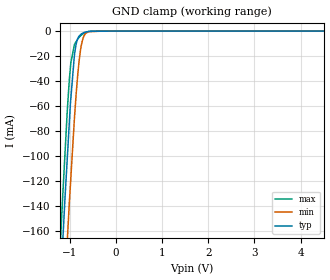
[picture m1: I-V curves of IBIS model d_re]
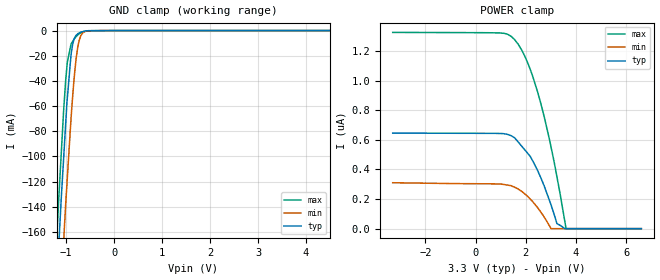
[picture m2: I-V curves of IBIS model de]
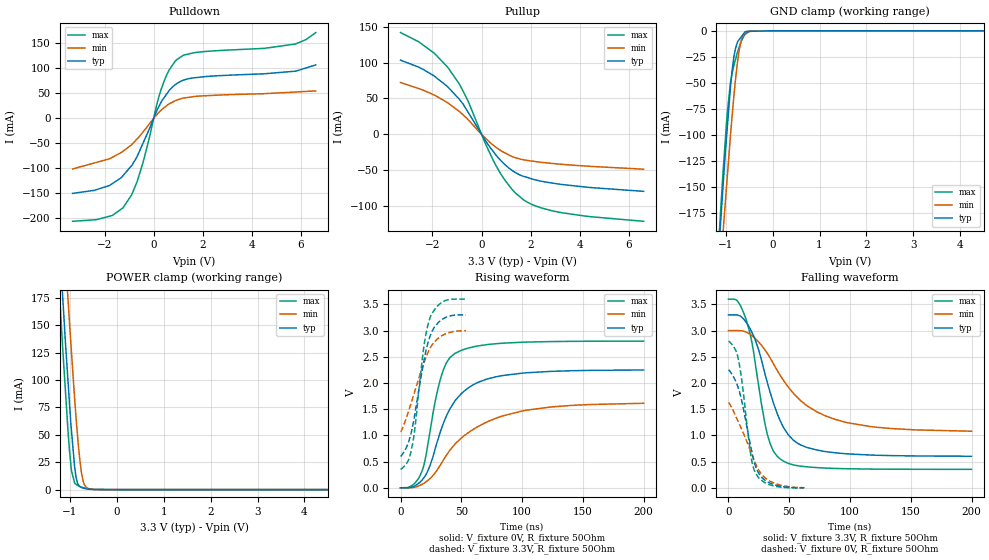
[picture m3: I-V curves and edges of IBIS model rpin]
|Texas Instruments Incorporated
| Robust Compact 3.3V-supply RS-485
| Marketing part#   Digital Voltage Range   Package-type   #pins
| SN65HVD72   3V - 3.6V   SOIC-8   8
[IBIS Ver]   3.2
[File name]   sn65hvd72.ibs
|SIMDE Ver   V3.0 - 201101 - RHL4 - Build 457
[File Rev]   1.0
[Date]   4/10/2012
[Source]
| Texas Instruments Incorporated.
| Analog-eLab Design Center, HPA
| 12500 TI Blvd
| Dallas, TX -75243
| e-mail: elab_scm_ibis@list.ti.com
[Notes]   Revision History:
| Rev 1.0: 4/10/2012
| - Initial version of the model
| - Model generated from simulations in TISPICE
| - Model matched to SPICE simulation
| - C_comp although listed in numerical order of value are
|   obtained from varying PVT conditions. For PVT conditions for
|   each specific value refer the buffer description under
|   respective [Model]. IBIS model user is responsible for using
|   appropriate C_comp to simulate for Signal Integrity.
|*  EXCEPTION:   *
|*  - For model d_re, there will be a leakage current in the GND   *
|*   clamp I-V Table because of the pullup on pad.   *
|*  - For model depin, there will be a leakage current in the POWER   *
|*   clamp I-V Table because of the pulldown on pad.   *
|*  - For model a_b, there will be a leakage current in the POWER clamp *
|*   I-V Table because of the pulldown resistor on pad and the resistor*
|*   network connected to pad and in the GND clamp I-V Table because of*
|*   the resistor network connected to pad.   *
|* -  For a_b_p and a_b_n models, pullup non-montonicity reflects true  *
|*   buffer behavior.   *
[Disclaimer]
| This model is designed as an aid for customers of Texas Instruments.
| TI and its licensors and suppliers make no warranties, either expressed
| or implied, with respect to this  model, including the warranties of
| merchantability or fitness for a particular purpose. The model is
| provided solely on an "as is" basis. The entire risk as to its quality
| and performance is with the customer.
[Copyright]
 (C) Copyright 2011 Texas Instruments Incorporated.All rights reserved.
|   SN65HVD72
[Component]   SN65HVD72D
[Manufacturer]   TI
[Package]   |8 SOIC-8  -  D package
|   typ   min   max
R_pkg   0.05625   0.05284   0.06331
L_pkg   2.58853nH   2.31916nH   3.13433nH
C_pkg   0.38513pF   0.35622pF   0.44246pF
[Pin]  signal_name   model_name   R_pin   L_pin   C_pin
1   R   rpin   0.06331   3.13433nH  0.44246pF
2   _RE   d_re   0.05416   2.35171nH  0.35866pF
3   DE   de   0.05284   2.31916nH  0.35622pF
4   D   d_re   0.05744   2.97557nH  0.43337pF
5   GND   gnd   0.02710   2.35557nH  0.47000pF
6   A   a_b_p   0.05477   2.37482nH  0.35995pF
7   B   a_b_n   0.05500   2.37562nH  0.36013pF
8   VCC   power   0.02780   2.39503nH  0.47300pF
[Diff_pin]   inv_pin   vdiff   tdelay_typ   tdelay_min   tdelay_max
6   7   0.2V   0   0   0
| Models and submodels in the file (5): d_re (Input), de (Input), rpin (3-state), a_b_p (I/O), a_b_n (I/O)
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|   d_re Model
[Model]   d_re
Model_type   Input
Vinl = 0.8
Vinh = 2
|   typ   min   max
|   (nom PVT)   (fast PVT)   (slow PVT)
C_comp   7.616e-13   7.309e-13   8.232e-13
| Where nom  PVT is Nominal Process, 3.3V, 27C
|   Fast PVT is Strong Process,  3.6V, -40C
|   Slow PVT is Weak Process,   3V, 125C
[Voltage Range]   3.3   3   3.6
|Ambient Temperature   25   125   -40
|Junction Temperature
[Temperature Range]   27   125   -40
[Power Clamp Reference]   3.3   3   3.6
[GND Clamp Reference]   0   0   0
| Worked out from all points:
|   GND clamp passes 1 mA (typ) near -0.67 V on its own axis
[GND Clamp]
|   Voltage   I(typ)   I(min)   I(max)
-3.3V     -1.936A    -1.939A    -1.964A
-1.188V   -195.6mA   -262.2mA   -159.6mA
-1.152V   -169.3mA   -236.4mA   -132.6mA
-1.105V   -136.2mA   -204.3mA   -100.5mA
-1.051V   -101.1mA   -166.9mA   -63.16mA
-975.6mV  -53.98mA   -117.4mA   -25.38mA
-897.6mV  -19.14mA   -69.83mA   -10.83mA
-858mV    -10mA      -49.27mA   -8.301mA
-792mV    -3.845mA   -22.53mA   -4.834mA
-693mV    -1.196mA   -3.958mA   -1.803mA
-285mV    -98.34uA   -1.769uA   -4.655uA
6.6V      0A         0A         0A
[POWER Clamp]
|   Voltage   I(typ)   I(min)   I(max)
-3.3V     0A         0A         0A
6.6V      0A         0A         0A
|   de Model
[Model]   de
Model_type   Input
Vinl = 0.8
Vinh = 2
|   typ   min   max
|   (nom PVT)   (fast PVT)   (slow PVT)
C_comp   7.616e-13   7.309e-13   8.232e-13
| Where nom  PVT is Nominal Process, 3.3V, 27C
|   Fast PVT is Strong Process,  3.6V, -40C
|   Slow PVT is Weak Process,   3V, 125C
[Voltage Range]   3.3   3   3.6
|Ambient Temperature   25   125   -40
|Junction Temperature
[Temperature Range]   27   125   -40
[Power Clamp Reference]   3.3   3   3.6
[GND Clamp Reference]   0   0   0
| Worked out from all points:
|   GND clamp passes 1 mA (typ) near -0.67 V on its own axis
[GND Clamp]
|   Voltage   I(typ)   I(min)   I(max)
-3.3V     -1.936A    -1.939A    -1.964A
-1.188V   -195.6mA   -262.2mA   -159.6mA
-1.152V   -169.3mA   -236.4mA   -132.6mA
-1.105V   -136.2mA   -204.3mA   -100.5mA
-1.051V   -101.1mA   -166.9mA   -63.16mA
-975.6mV  -53.98mA   -117.4mA   -25.38mA
-897.6mV  -19.14mA   -69.83mA   -10.83mA
-858mV    -10mA      -49.27mA   -8.301mA
-792mV    -3.845mA   -22.53mA   -4.834mA
-693mV    -1.196mA   -3.959mA   -1.803mA
-285mV    -98uA      -1.603uA   -3.947uA
6.6V      0A         0A         0A
[POWER Clamp]
|   Voltage   I(typ)   I(min)   I(max)
-3.3V     645nA      310.1nA    1.325uA
939.6mV   642.6nA    301.8nA    1.322uA
1.422V    626.9nA    289.4nA    1.298uA
1.685V    587.5nA    268.5nA    1.248uA
1.948V    534.5nA    236.2nA    1.169uA
2.168V    490.1nA    201.3nA    1.079uA
2.473V    391.4nA    141.5nA    921.2nA
2.736V    286.6nA    77.39nA    753.7nA
3.003V    161.7nA    0A         553nA
3.241V    34.27nA    0A         349.4nA
3.604V    0A         0A         0A
6.6V      0A         0A         0A
|   rpin Model
[Model]   rpin
Model_type   3-state
Polarity   Non-Inverting
Vmeas = 1.65
Vref = 1.65
Cref = 2pF
Rref = 50
|   typ   min   max
|   (nom PVT)   (fast PVT)   (slow PVT)
C_comp   2.762e-12   2.415e-12   2.953e-12
|ON state : BUFFER OUTPUT TURNED HIGH
|C_comp   2.762e-12   2.415e-12   2.953e-12
|OFF state: BUFFER IN HIGH IMPEDANCE
|C_comp   2.507e-12   2.233e-12   2.622e-12
| Where nom  PVT is Nominal Process, 3.3V, 27C
|   Fast PVT is Strong Process,  3.6V, -40C
|   Slow PVT is Weak Process,   3V, 125C
[Voltage Range]   3.3   3   3.6
|Ambient Temperature   25   125   -40
|Junction Temperature
[Temperature Range]   27   125   -40
[Pullup Reference]   3.3   3   3.6
[Pulldown Reference]   0   0   0
[Power Clamp Reference]   3.3   3   3.6
[GND Clamp Reference]   0   0   0
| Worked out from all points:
|   slope of the pulldown table from 0 to 0.495 V, typ, clamps not added: 10.7 ohm
|   slope of the pullup table from 0 to 0.495 V, typ, clamps not added: 20.1 ohm
|   GND clamp passes 1 mA (typ) near -0.58 V on its own axis
|   POWER clamp passes 1 mA (typ) near -0.68 V on its own axis
|   falling waveform, V_fixture 3.3V, R_fixture 50Ohm: 20-80 % time 22.6ns typ, 41.2ns min, 14.6ns max; typ from 3.3 V to 0.603 V
|   rising waveform, V_fixture 0V, R_fixture 50Ohm: 20-80 % time 25.5ns typ, 45ns min, 14.6ns max; typ from 0 V to 2.25 V
|   rising waveform, V_fixture 3.3V, R_fixture 50Ohm: 20-80 % time 12.8ns typ, 16.7ns min, 10ns max; typ from 0.601 V to 3.3 V
|   falling waveform, V_fixture 0V, R_fixture 50Ohm: 20-80 % time 12.3ns typ, 17.9ns min, 9.02ns max; typ from 2.25 V to 0 V
[Pulldown]
|   Voltage   I(typ)   I(min)   I(max)
-3.3V     -149.9mA   -101.1mA   -205.7mA
-1.681V   -130.4mA   -77.73mA   -193.9mA
-1.249V   -114.5mA   -65.67mA   -178.9mA
-896.4mV  -94.5mA    -52.62mA   -153mA
-673.2mV  -76.17mA   -41.18mA   -126.5mA
-428.4mV  -49.17mA   -26.94mA   -87.39mA
306mV     32.4mA     16.57mA    58.12mA
633.6mV   55.83mA    28.96mA    96.76mA
939.6mV   69.38mA    36.44mA    117.2mA
1.706V    81.24mA    43.83mA    131.5mA
5.771V    94.13mA    52.57mA    148.4mA
6.6V      106.7mA    54.76mA    171.3mA
[GND Clamp]
|   Voltage   I(typ)   I(min)   I(max)
-3.3V     -1.902A    -1.839A    -1.974A
-1.162V   -220.6mA   -261.9mA   -213.2mA
-1.066V   -156mA     -200mA     -142.2mA
-1.041V   -139.5mA   -184.6mA   -126.3mA
-968.4mV  -94.65mA   -142mA     -79.83mA
-896.4mV  -53.3mA    -99.73mA   -49.1mA
-825mV    -25.05mA   -62.73mA   -33.45mA
-714mV    -8.529mA   -19.14mA   -15.82mA
-648mV    -4.59mA    -6.136mA   -8.088mA
-590.7mV  -1.17mA    -1.793mA   -3.636mA
-439.2mV  -366.3uA   -451.5uA   -96.91uA
6.6V      0A         0A         0A
[Pullup]
|   Voltage   I(typ)   I(min)   I(max)
-3.3V     103.4mA    72.23mA    141.8mA
-2.56V    93.59mA    63.81mA    129mA
-1.926V   81.19mA    54.79mA    113mA
-1.375V   66.15mA    43.89mA    93.39mA
-896.4mV  48.62mA    31.69mA    69.68mA
-572.4mV  32.23mA    21.44mA    48.14mA
172.8mV   -9.472mA   -5.689mA   -14.19mA
633.6mV   -30.76mA   -19.2mA    -46.34mA
1.246V    -50.27mA   -30.87mA   -76.8mA
1.706V    -58.35mA   -35.31mA   -91.08mA
3.287V    -69.84mA   -41.73mA   -109.2mA
6.6V      -79.34mA   -48.49mA   -121mA
[POWER Clamp]
|   Voltage   I(typ)   I(min)   I(max)
-3.3V     1.851A     1.898A     1.834A
-1.274V   263.2mA    340.2mA    218.9mA
-1.152V   176mA      252mA      128.8mA
-1.037V   97.77mA    172.5mA    52.17mA
-964.8mV  53.62mA    125.4mA    17.12mA
-897.6mV  20.44mA    82.88mA    5.965mA
-867.9mV  11.43mA    66.12mA    4.84mA
-816mV    4.319mA    39.38mA    3.473mA
-745.8mV  1.73mA     13.98mA    2.211mA
-660mV    790uA      2.331mA    1.324mA
-486mV    190.9uA    98.8uA     38.01uA
6.6V      0A         0A         0A
[Ramp]
R_load = 50
|   typ   min   max
dV/dt_r   1.34939/2.5469e-08   0.967996/4.48304e-08   1.6794/1.46144e-08
dV/dt_f   1.61822/2.25372e-08   1.15176/4.11029e-08   1.94808/1.45548e-08
[Falling Waveform]
V_fixture = 3.3V
V_fixture_min = 3V
V_fixture_max = 3.6V
R_fixture = 50Ohm
|   Time   V(typ)   V(min)   V(max)
0s        3.3V       3V         3.6V
7.64ns    3.295V     3V         3.56V
14.66ns   3.156V     2.971V     3.202V
19.4ns    2.963V     2.9V       2.763V
31.94ns   2.013V     2.568V     1.027V
36.72ns   1.641V     2.379V     711.5mV
43.84ns   1.218V     2.099V     530mV
57.76ns   839.4mV    1.699V     420mV
88.84ns   666.1mV    1.298V     369.7mV
200ns     603mV      1.08V      353.2mV
[Rising Waveform]
V_fixture = 0V
V_fixture_min = 0V
V_fixture_max = 0V
R_fixture = 50Ohm
|   Time   V(typ)   V(min)   V(max)
0s        613pV      31.56nV    241.3pV
9.9ns     17.78mV    4.805mV    51.09mV
17.42ns   141.7mV    62.83mV    306.1mV
24.28ns   425.8mV    177.3mV    1.076V
32.74ns   1.068V     434.2mV    2.069V
37.94ns   1.381V     629.3mV    2.391V
44.78ns   1.658V     833.6mV    2.564V
63.9ns    2.014V     1.172V     2.708V
100.1ns   2.188V     1.466V     2.778V
200ns     2.249V     1.613V     2.799V
[Rising Waveform]
V_fixture = 3.3V
V_fixture_min = 3V
V_fixture_max = 3.6V
R_fixture = 50Ohm
|   Time   V(typ)   V(min)   V(max)
0s        601.3mV    1.07V      353mV
6.48ns    865.5mV    1.453V     527.3mV
9.72ns    1.147V     1.692V     815.7mV
12.26ns   1.477V     1.881V     1.223V
18.86ns   2.374V     2.358V     2.639V
21.46ns   2.669V     2.52V      2.997V
24.84ns   2.925V     2.687V     3.279V
29.46ns   3.11V      2.823V     3.446V
35.46ns   3.232V     2.921V     3.559V
53.8ns    3.3V       2.999V     3.6V
[Falling Waveform]
V_fixture = 0V
V_fixture_min = 0V
V_fixture_max = 0V
R_fixture = 50Ohm
|   Time   V(typ)   V(min)   V(max)
0s        2.252V     1.625V     2.8V
5.48ns    2.059V     1.395V     2.647V
8.5ns     1.877V     1.241V     2.415V
11.72ns   1.576V     1.074V     1.918V
14.68ns   1.231V     909mV      1.302V
18.68ns   751.4mV    669.7mV    576.9mV
21.56ns   462.8mV    502.1mV    317.7mV
27ns      207.8mV    267.8mV    150.4mV
34.04ns   90.81mV    128.9mV    57.95mV
62.32ns   185.3uV    2.383mV    41.92uV
